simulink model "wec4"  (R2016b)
settings: Solver=ode4  StartTime=0  StopTime=1000  FixedStep=0.005  MaxStep=0.005  RelTol=1e-3  EnableMultiTasking=on
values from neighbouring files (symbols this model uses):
  arAdaptiveLawData = 1/2*zModelSimple.zModelPto.arFreq.*     zModelSimple.zModelPto.arMagnitude./     cos(zModelSimple.zModelPto.arPhase*pi/180+pi/2)    [IMPACT_Control.m]
  arAdaptiveLawDataX = 1/2*zModelSimpleX.zModelPto.arFreq.*         zModelSimpleX.zModelPto.arMagnitude./         cos(zModelSimpleX.zModelPto.arPhase*pi/180+pi/2)    [IMPACT_Control.m]
  arControllerRampGain = [0,0,1,1]    [IMPACT_Control.m]
  arControllerRampTime = [0 rStartRampTime rStartRampTime+rRampTimeLength 8000]    [IMPACT_Control.m]
  arEkfInitialisation = zeros(1,11)    [IMPACT_Control.m]
  arEkfInitialisationX = zeros(1,11)    [IMPACT_Control.m]
  arFrequency = zModelSimple.zModelPto.arFreq    [IMPACT_Control.m]
  arFrequencyRange = zModelSimple.zModelPto.arFreq    [IMPACT_Control.m]
  arFrequencyX = zModelSimpleX.zModelPto.arFreq    [IMPACT_Control.m]
  arImpedance = 1./zModelSimple.zModelPto.arMagnitude./zModelSimple.zModelPto.arFreq    [IMPACT_Control.m]
  arImpedanceX = 1./zModelSimpleX.zModelPto.arMagnitude./zModelSimpleX.zModelPto.arFreq    [IMPACT_Control.m]
  CentralPTOPreload = -1.6113e+07    (= -16113000)    [wecSimInputFile.m]
  F1 = [4.243 2.375 -12.243]    [wecSimInputFile.m]
  F2 = [4.243 -2.375 -12.243]    [wecSimInputFile.m]
  F3 = [-4.243 -2.375 -12.243]    [wecSimInputFile.m]
  F4 = [-4.243 2.375 -12.243]    [wecSimInputFile.m]
  FC = [0 0 -14]    [wecSimInputFile.m]
  iAdaptiveDamping = 0    [wec4IMPACT_Project.m]    (also in IMPACT_Control.m = handles.iAdaptiveDamping; wec1_IMPACT_Project.m; wec2_IMPACT_Project.m; wec3_IMPACT_Project.m)
  iControlType = 2    [wec4IMPACT_Project.m]    (also in IMPACT_Control.m = handles.iControlType; wec1_IMPACT_Project.m = 1; wec2_IMPACT_Project.m = 1; wec3_IMPACT_Project.m = 1)
  iPtoPositionConstraint = 1    [wec4IMPACT_Project.m]    (also in IMPACT_Control.m = handles.iPtoPositionConstraint; wec1_IMPACT_Project.m = 0; wec2_IMPACT_Project.m; wec3_IMPACT_Project.m)
  iSensorNoise = 0    [IMPACT_Control.m]
  m = m+1    (= 2)    [checkParamFile.m]
  PTOrotation = atan((T1(2)-F1(2))/(T1(1)-F1(1)))    [wecSimInputFile.m]
  rCogFloater = -8    [wec4_IMPACT_Model.m]    (also in paramInitial.m = get( handles.edit_rCogFloater, 'String' ); wec1_IMPACT_Model.m = -18; wec2_IMPACT_Model.m = -8.5; wec3_IMPACT_Model.m = -0.7)
  rCogSpar = -36.6    [wec4_IMPACT_Model.m]    (also in paramInitial.m = get( handles.edit_rCogSpar, 'String' ); wec3_IMPACT_Model.m = -21.3; wec3_IMPACT_Model2.m = -21.3)
  rDisplacementLimit = 10.000000    (= 10)    [wec4IMPACT_Project.m]    (also in IMPACT_Control.m = getValue(handles.edit_displacementLimit); wec1_IMPACT_Project.m; wec2_IMPACT_Project.m; wec3_IMPACT_Project.m = 3)
  rDisplacementLimitX = 10.000000    (= 10)    [wec4IMPACT_Project.m]    (also in IMPACT_Control.m = getValue(handles.edit_displacementLimitX); wec1_IMPACT_Project.m = 0; wec2_IMPACT_Project.m; wec3_IMPACT_Project.m = 0)
  rGainForAntiWIndUp = tfControllerDiscrete.rGain    [IMPACT_Control.m]
  rGainForAntiWIndUpX = tfControllerXDiscrete.rGain    [IMPACT_Control.m]
  rMaxForcePto = 300000000.000000    (= 300000000)    [wec4IMPACT_Project.m]    (also in IMPACT_Control.m = getValue(handles.edit_maxForcePto); wec1_IMPACT_Project.m = 1e+15; wec2_IMPACT_Project.m = 1e+15; wec3_IMPACT_Project.m = 1000000000)
  rMinForcePto = -300000000.000000    (= -300000000)    [wec4IMPACT_Project.m]    (also in IMPACT_Control.m = getValue(handles.edit_minForcePto); wec1_IMPACT_Project.m = -1e+15; wec2_IMPACT_Project.m = -1e+15; wec3_IMPACT_Project.m = -1000000000)
  rMooringX = 20000    [wec4_IMPACT_Model.m]    (also in paramInitial.m = get( handles.edit_rMooringX, 'String' ); wec3_IMPACT_Model.m = 10000; wec3_IMPACT_Model2.m = 10000)
  rMooringZ = 10000    [wec4_IMPACT_Model.m]    (also in paramInitial.m = get( handles.edit_rMooringZ, 'String' ); wec3_IMPACT_Model.m = 0; wec3_IMPACT_Model2.m = 0)
  rOutputSampleTime = 0.010000    (= 0.01)    [wec4IMPACT_Project.m]    (also in IMPACT_Control.m = getValue(handles.edit_outputSampleTime); wec1_IMPACT_Project.m; wec2_IMPACT_Project.m; wec3_IMPACT_Project.m)
  rPassiveDampingGain = -604830.000000    (= -604830)    [wec4IMPACT_Project.m]    (also in IMPACT_Control.m = getValue(handles.edit_gainPLD); wec1_IMPACT_Project.m = -214018.1537; wec2_IMPACT_Project.m = -1948070; wec3_IMPACT_Project.m = -519390)
  rPassiveDampingGainX = -278660.000000    (= -278660)    [wec4IMPACT_Project.m]    (also in IMPACT_Control.m = getValue(handles.edit_gainPLDX); wec1_IMPACT_Project.m = 0; wec2_IMPACT_Project.m = 0; wec3_IMPACT_Project.m = 0)
  rTetherPretension = 1.6113e+07    (= 16113000)    [wec4_IMPACT_Model.m]    (also in paramInitial.m = get( handles.edit_rTetherPretension, 'String' ); wec3_IMPACT_Model.m = 0; wec3_IMPACT_Model2.m = 0)
  rTetherSpring = 500000    [wec4_IMPACT_Model.m]    (also in paramInitial.m = get( handles.edit_rTetherSpring, 'String' ); wec3_IMPACT_Model.m = 0; wec3_IMPACT_Model2.m = 0)
  rUpperFrequencyLimit = EKFFloater.upperFreq    [IMPACT_Control.m]
  rXf = 4.243    [wec4AdditionalParams.m]
  rXs = 16.075    [wec4AdditionalParams.m]
  rYf = 2.375    [wec4AdditionalParams.m]
  rYs = 16.075    [wec4AdditionalParams.m]
  rZf = 4.243    [wec4AdditionalParams.m]
  rZs = 2.4350    (= 2.435)    [wec4AdditionalParams.m]
  rZTetherF = 6    [wec4AdditionalParams.m]
  rZTetherS = 2.4350    (= 2.435)    [wec4AdditionalParams.m]
  s = tf('s')    [wec4_IMPACT_Model.m]    (also in IMPACT_Control.m; wec1_IMPACT_Model.m; wec2_IMPACT_Model.m; wec3_IMPACT_Model.m)
  SidePTO1Preload = PreloadPTOCorner    (= 0)    [wecSimInputFile.m]
  SidePTO2Preload = PreloadPTOCorner    (= 0)    [wecSimInputFile.m]
  SidePTO3Preload = PreloadPTOCorner    (= 0)    [wecSimInputFile.m]
  SidePTO4Preload = PreloadPTOCorner    (= 0)    [wecSimInputFile.m]
  simu = simulationClass()    [wecSimInputFile.m]
  T1 = [16.075 16.075 -34.165]    [wecSimInputFile.m]
  T2 = [16.075 -16.075 -34.165]    [wecSimInputFile.m]
  T3 = [-16.075 -16.075 -34.165]    [wecSimInputFile.m]
  T4 = [-16.075 16.075 -34.165]    [wecSimInputFile.m]
  TC = [0 0 -34.165]    [wecSimInputFile.m]
  waves = waveClass('irregular')    [wecSimInputFile.m]
  Z = magPhaseToComplex(zModelTf)    [IMPACT_Control.m]
undefined symbols (not defined in the file or in its folder): arControllerDiscreteDen, arControllerDiscreteNum, arControllerDiscreteXDen, arControllerDiscreteXNum, arExcForceFloaterDen, arExcForceFloaterNum, arExcForceFloaterXDen, arExcForceFloaterXNum, arExcForceSparDen, arExcForceSparNum, arExcForceSparXDen, arExcForceSparXNum, arFexcFloaterDen, arFexcFloaterNum, arFexcFloaterXDen, arFexcFloaterXNum, arFexcSparDen, arFexcSparNum, arFexcSparXDen, arFexcSparXNum, Body, body, constraint, CTTime, deg, Elements, geometry, IRKB, kg, lenJ, mooring, N, pto, rAccelerationGainFloater, rAccelerationGainFloaterX, rAccelerationGainSpar, rAccelerationGainSparX, rad, rBuoyancyGainFloater, rBuoyancyGainFloaterX, rBuoyancyGainSpar, rBuoyancyGainSparX, rDampingGainFloater, rDampingGainFloaterX, rDampingGainSpar, rDampingGainSparX, Rigid, rMaxFocePto, wec4_float, wec4_reactor, WECSim_Lib, X, Y
libraries: nesl_utility x380, sm_lib x170, vrlib x91, simulink x12, WECSim_Lib x4
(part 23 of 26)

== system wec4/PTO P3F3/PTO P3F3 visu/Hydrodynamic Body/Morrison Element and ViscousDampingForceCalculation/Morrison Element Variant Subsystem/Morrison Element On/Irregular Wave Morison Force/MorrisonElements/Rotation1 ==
  rot1 : Inport
  rot2 : Inport  Port=2
  rot3 : Inport  Port=3
  2 : Product
  3 : Product  Inputs=3
  7 : Product
  8 : Product  Inputs=3
  Combine : Concatenate  NumInputs=3  Mode=Multidimensional array  ConcatenateDimension=2
  Trigonometric Function{,1..2,6,9,11} (6 alike) : Trigonometry  Operator=cos
  Trigonometric Function{3..5,7..8,10} (6 alike) : Trigonometry
  rot11 : Product
  rot12 : Sum
  rot13 : Sum  Inputs=+-
  rot[1,1-3] : Outport
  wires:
  rot13/1 -> Combine/3
  8/1 -> rot13/2
  7/1 -> rot13/1
  Trigonometric Function11/1 -> 8/3
  Trigonometric Function10/1 -> 8/2
  Trigonometric Function9/1 -> 8/1
  Trigonometric Function8/1 -> 7/2
  Trigonometric Function7/1 -> 7/1
  rot1/1 -> Trigonometric Function7/1, Trigonometric Function9/1, Trigonometric Function4/1, Trigonometric Function2/1
  rot3/1 -> Trigonometric Function8/1, Trigonometric Function11/1, Trigonometric Function6/1, Trigonometric Function3/1, Trigonometric Function1/1
  rot2/1 -> Trigonometric Function10/1, Trigonometric Function5/1, Trigonometric Function/1
  Combine/1 -> rot[1,1-3]/1
  rot12/1 -> Combine/2
  3/1 -> rot12/2
  2/1 -> rot12/1
  Trigonometric Function6/1 -> 3/3
  Trigonometric Function5/1 -> 3/2
  Trigonometric Function4/1 -> 3/1
  Trigonometric Function3/1 -> 2/2
  Trigonometric Function2/1 -> 2/1
  rot11/1 -> Combine/1
  Trigonometric Function1/1 -> rot11/2
  Trigonometric Function/1 -> rot11/1

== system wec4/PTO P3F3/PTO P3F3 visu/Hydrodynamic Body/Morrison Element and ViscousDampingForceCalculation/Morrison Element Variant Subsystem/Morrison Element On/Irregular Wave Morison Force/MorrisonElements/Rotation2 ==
  rot1 : Inport
  rot2 : Inport  Port=2
  rot3 : Inport  Port=3
  2 : Product
  3 : Product  Inputs=3
  7 : Product
  8 : Product  Inputs=3
  Combine : Concatenate  NumInputs=3  Mode=Multidimensional array  ConcatenateDimension=2
  Gain : Gain  Gain=-1
  Trigonometric Function{,2..3,8..9} (5 alike) : Trigonometry  Operator=cos
  Trigonometric Function{1,4..7,10..11} (7 alike) : Trigonometry
  rot11 : Product
  rot12 : Sum  Inputs=+-
  rot13 : Sum
  rot[2,1-3] : Outport
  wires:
  Gain/1 -> rot11/1
  rot13/1 -> Combine/3
  8/1 -> rot13/2
  7/1 -> rot13/1
  Trigonometric Function11/1 -> 8/3
  Trigonometric Function10/1 -> 8/2
  Trigonometric Function9/1 -> 8/1
  Trigonometric Function8/1 -> 7/2
  Trigonometric Function7/1 -> 7/1
  rot1/1 -> Trigonometric Function7/1, Trigonometric Function9/1, Trigonometric Function4/1, Trigonometric Function2/1
  rot3/1 -> Trigonometric Function8/1, Trigonometric Function11/1, Trigonometric Function6/1, Trigonometric Function3/1, Trigonometric Function1/1
  rot2/1 -> Trigonometric Function10/1, Trigonometric Function5/1, Trigonometric Function/1
  Combine/1 -> rot[2,1-3]/1
  rot12/1 -> Combine/2
  3/1 -> rot12/2
  2/1 -> rot12/1
  Trigonometric Function6/1 -> 3/3
  Trigonometric Function5/1 -> 3/2
  Trigonometric Function4/1 -> 3/1
  Trigonometric Function3/1 -> 2/2
  Trigonometric Function2/1 -> 2/1
  rot11/1 -> Combine/1
  Trigonometric Function1/1 -> rot11/2
  Trigonometric Function/1 -> Gain/1

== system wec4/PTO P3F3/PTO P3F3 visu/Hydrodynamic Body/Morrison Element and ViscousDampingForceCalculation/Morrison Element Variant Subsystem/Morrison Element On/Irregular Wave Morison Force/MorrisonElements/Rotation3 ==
  rot1 : Inport
  rot2 : Inport  Port=2
  2 : Product
  7 : Product
  Combine : Concatenate  NumInputs=3  Mode=Multidimensional array  ConcatenateDimension=2
  Gain1 : Gain  Gain=-1
  TrigFun1 : Trigonometry
  TrigFun2 : Trigonometry
  TrigFun3 : Trigonometry  Operator=cos
  TrigFun4 : Trigonometry  Operator=cos
  TrigFun5 : Trigonometry  Operator=cos
  rot[3,1-3] : Outport
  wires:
  Gain1/1 -> 2/1
  TrigFun2/1 -> Gain1/1
  7/1 -> Combine/3
  rot1/1 -> TrigFun4/1, TrigFun2/1
  TrigFun5/1 -> 7/2
  TrigFun4/1 -> 7/1
  rot2/1 -> TrigFun1/1, TrigFun3/1, TrigFun5/1
  Combine/1 -> rot[3,1-3]/1
  2/1 -> Combine/2
  TrigFun3/1 -> 2/2
  TrigFun1/1 -> Combine/1

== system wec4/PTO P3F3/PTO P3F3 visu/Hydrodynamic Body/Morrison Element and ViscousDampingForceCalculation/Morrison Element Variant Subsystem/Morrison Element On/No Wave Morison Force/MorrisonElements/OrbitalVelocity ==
  Disp : Inport
  Time : Inport  Port=2
  AmpMerge : Merge
  Applied Ramp Function : Subsystem  TreatAsAtomicUnit=on
  Disp-slx : Selector  InputPortWidth=3  IndexOptions=Index vector (dialog)  Indices=[1]  OutputSizes=1
  Disp-sly : Selector  InputPortWidth=3  IndexOptions=Index vector (dialog)  Indices=[2]  OutputSizes=1
  Disp-slz : Selector  InputPortWidth=3  IndexOptions=Index vector (dialog)  Indices=[3]  OutputSizes=1
  Gain : Gain  Gain=pi/180
  Gravity : Constant  Value=simu.g
  HorizHead : Trigonometry  Operator=cos
  Horizontal-x,y : Trigonometry  Operator=cos
  Horizontal-z : Trigonometry  Operator=cosh
  No Ramp Function : Subsystem  TreatAsAtomicUnit=on
  Ramp : If  NumInputs=2  IfExpression=u1 < u2
  Ramp Function Time : Constant  Value=simu.rampTime
  VertHead : Trigonometry
  Vertical-x,y : Trigonometry
  Vertical-z : Trigonometry  Operator=sinh
  WaterDepth : Constant  Value=waves.waterDepth
  WaveAmp : Constant  Value=waves.A(1,:)
  WaveFreq : Constant  Value=waves.w(1,:)
  WaveHeading : Constant  Value=waves.waveDir
  WaveNumber : Constant  Value=waves.k(1,:)
  X-A : Gain  Gain=-1
  Y-A : Gain  Gain=-1
  Y-V : Gain  Gain=-1
  Z-A : Gain  Gain=-1
  cosh : Trigonometry  Operator=cosh
  cosh*cos : Product  Inputs=**
  cosh*sin : Product  Inputs=**
  cosh/coshkh : Product  Inputs=*/
  k(xcos + ysin) : Sum
  k*h : Product
  k*x*cos(beta) : Product  Inputs=3
  k*y*sin(beta) : Product  Inputs=3
  k*z : Product
  sigma*t : Product
  sincos : Sum  Inputs=-+
  sinh*cos : Product  Inputs=**
  sinh*sin : Product  Inputs=**
  sinh/coshkh : Product  Inputs=*/
  sinhcosh : Sum
  u-Accel : Product  Inputs=*****
  u-Vel : Product  Inputs=****/*
  u-Vel1 : Product  Inputs=****/*
  v-Accel : Product  Inputs=*****
  w-Accel : Product  Inputs=****
  w-Vel : Product  Inputs=****/
  u-V : Outport
  w-V : Outport  Port=2
  u-A : Outport  Port=3
  w-A : Outport  Port=4
  v-V : Outport  Port=5
  v-A : Outport  Port=6
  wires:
  v-Accel/1 -> v-A/1
  Y-A/1 -> v-Accel/1
  u-Vel/1 -> u-V/1
  u-Vel1/1 -> v-V/1
  k(xcos + ysin)/1 -> sincos/1
  k*x*cos(beta)/1 -> k(xcos + ysin)/1
  k*y*sin(beta)/1 -> k(xcos + ysin)/2
  VertHead/1 -> v-Accel/5, u-Vel1/6, k*y*sin(beta)/1
  HorizHead/1 -> k*x*cos(beta)/1, u-Vel/6, u-Accel/5
  Disp-slx/1 -> k*x*cos(beta)/2
  Gain/1 -> VertHead/1, HorizHead/1
  WaveHeading/1 -> Gain/1
  WaveAmp/1 -> No Ramp Function/1(Ain), Applied Ramp Function/1(Ain)
  WaveFreq/1 -> sigma*t/1, u-Vel/5, u-Vel1/5, w-Vel/5
  Disp-slz/1 -> k*z/1
  Applied Ramp Function/1(Aout) -> AmpMerge/1
  No Ramp Function/1(Aout) -> AmpMerge/2
  Time/1 -> sigma*t/2, Ramp/1
  Ramp/1 -> Applied Ramp Function/Action
  Ramp/2 -> No Ramp Function/Action
  Ramp Function Time/1 -> Ramp/2
  sinh*cos/1 -> Z-A/1
  cosh*sin/1 -> X-A/1, Y-A/1
  w-Accel/1 -> w-A/1
  u-Accel/1 -> u-A/1
  w-Vel/1 -> w-V/1
  Z-A/1 -> w-Accel/1
  X-A/1 -> u-Accel/1
  Y-V/1 -> w-Vel/1
  sinh*sin/1 -> Y-V/1
  Gravity/1 -> u-Vel/3, u-Vel1/3, u-Accel/3, w-Accel/3, v-Accel/3, w-Vel/3
  AmpMerge/1 -> u-Vel/2, u-Vel1/2, u-Accel/2, v-Accel/2, w-Accel/2, w-Vel/2
  cosh*cos/1 -> u-Vel/1, u-Vel1/1
  Disp-sly/1 -> k*y*sin(beta)/2
  cosh/coshkh/1 -> cosh*sin/2, cosh*cos/2
  Horizontal-x,y/1 -> cosh*cos/1, sinh*cos/1
  sinh/coshkh/1 -> sinh*sin/2, sinh*cos/2
  Vertical-x,y/1 -> sinh*sin/1, cosh*sin/1
  Vertical-z/1 -> sinh/coshkh/1
  cosh/1 -> cosh/coshkh/2, sinh/coshkh/2
  Horizontal-z/1 -> cosh/coshkh/1
  sinhcosh/1 -> Horizontal-z/1, Vertical-z/1
  k*h/1 -> sinhcosh/2, cosh/1
  k*z/1 -> sinhcosh/1
  sincos/1 -> Horizontal-x,y/1, Vertical-x,y/1
  sigma*t/1 -> sincos/2
  WaterDepth/1 -> k*h/1
  WaveNumber/1 -> u-Vel/4, u-Vel1/4, u-Accel/4, w-Accel/4, v-Accel/4, w-Vel/4, k*x*cos(beta)/3, k*y*sin(beta)/3, k*z/2, k*h/2
  Disp/1 -> Disp-slx/1, Disp-sly/1, Disp-slz/1

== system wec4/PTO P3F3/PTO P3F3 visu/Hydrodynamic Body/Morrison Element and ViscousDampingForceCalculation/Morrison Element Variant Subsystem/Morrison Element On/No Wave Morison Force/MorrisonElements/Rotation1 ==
  rot1 : Inport
  rot2 : Inport  Port=2
  rot3 : Inport  Port=3
  2 : Product
  3 : Product  Inputs=3
  7 : Product
  8 : Product  Inputs=3
  Combine : Concatenate  NumInputs=3  Mode=Multidimensional array  ConcatenateDimension=2
  Trigonometric Function{,1..2,6,9,11} (6 alike) : Trigonometry  Operator=cos
  Trigonometric Function{3..5,7..8,10} (6 alike) : Trigonometry
  rot11 : Product
  rot12 : Sum
  rot13 : Sum  Inputs=+-
  rot[1,1-3] : Outport
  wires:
  rot13/1 -> Combine/3
  8/1 -> rot13/2
  7/1 -> rot13/1
  Trigonometric Function11/1 -> 8/3
  Trigonometric Function10/1 -> 8/2
  Trigonometric Function9/1 -> 8/1
  Trigonometric Function8/1 -> 7/2
  Trigonometric Function7/1 -> 7/1
  rot1/1 -> Trigonometric Function7/1, Trigonometric Function9/1, Trigonometric Function4/1, Trigonometric Function2/1
  rot3/1 -> Trigonometric Function8/1, Trigonometric Function11/1, Trigonometric Function6/1, Trigonometric Function3/1, Trigonometric Function1/1
  rot2/1 -> Trigonometric Function10/1, Trigonometric Function5/1, Trigonometric Function/1
  Combine/1 -> rot[1,1-3]/1
  rot12/1 -> Combine/2
  3/1 -> rot12/2
  2/1 -> rot12/1
  Trigonometric Function6/1 -> 3/3
  Trigonometric Function5/1 -> 3/2
  Trigonometric Function4/1 -> 3/1
  Trigonometric Function3/1 -> 2/2
  Trigonometric Function2/1 -> 2/1
  rot11/1 -> Combine/1
  Trigonometric Function1/1 -> rot11/2
  Trigonometric Function/1 -> rot11/1

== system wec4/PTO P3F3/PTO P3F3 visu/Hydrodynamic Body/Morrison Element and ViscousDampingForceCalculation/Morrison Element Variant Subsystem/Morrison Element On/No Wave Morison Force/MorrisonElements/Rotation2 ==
  rot1 : Inport
  rot2 : Inport  Port=2
  rot3 : Inport  Port=3
  2 : Product
  3 : Product  Inputs=3
  7 : Product
  8 : Product  Inputs=3
  Combine : Concatenate  NumInputs=3  Mode=Multidimensional array  ConcatenateDimension=2
  Gain : Gain  Gain=-1
  Trigonometric Function{,2..3,8..9} (5 alike) : Trigonometry  Operator=cos
  Trigonometric Function{1,4..7,10..11} (7 alike) : Trigonometry
  rot11 : Product
  rot12 : Sum  Inputs=+-
  rot13 : Sum
  rot[2,1-3] : Outport
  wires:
  Gain/1 -> rot11/1
  rot13/1 -> Combine/3
  8/1 -> rot13/2
  7/1 -> rot13/1
  Trigonometric Function11/1 -> 8/3
  Trigonometric Function10/1 -> 8/2
  Trigonometric Function9/1 -> 8/1
  Trigonometric Function8/1 -> 7/2
  Trigonometric Function7/1 -> 7/1
  rot1/1 -> Trigonometric Function7/1, Trigonometric Function9/1, Trigonometric Function4/1, Trigonometric Function2/1
  rot3/1 -> Trigonometric Function8/1, Trigonometric Function11/1, Trigonometric Function6/1, Trigonometric Function3/1, Trigonometric Function1/1
  rot2/1 -> Trigonometric Function10/1, Trigonometric Function5/1, Trigonometric Function/1
  Combine/1 -> rot[2,1-3]/1
  rot12/1 -> Combine/2
  3/1 -> rot12/2
  2/1 -> rot12/1
  Trigonometric Function6/1 -> 3/3
  Trigonometric Function5/1 -> 3/2
  Trigonometric Function4/1 -> 3/1
  Trigonometric Function3/1 -> 2/2
  Trigonometric Function2/1 -> 2/1
  rot11/1 -> Combine/1
  Trigonometric Function1/1 -> rot11/2
  Trigonometric Function/1 -> Gain/1

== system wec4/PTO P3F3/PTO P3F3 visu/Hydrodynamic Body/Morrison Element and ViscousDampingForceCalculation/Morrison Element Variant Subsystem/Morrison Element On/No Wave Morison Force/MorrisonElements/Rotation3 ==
  rot1 : Inport
  rot2 : Inport  Port=2
  2 : Product
  7 : Product
  Combine : Concatenate  NumInputs=3  Mode=Multidimensional array  ConcatenateDimension=2
  Gain1 : Gain  Gain=-1
  TrigFun1 : Trigonometry
  TrigFun2 : Trigonometry
  TrigFun3 : Trigonometry  Operator=cos
  TrigFun4 : Trigonometry  Operator=cos
  TrigFun5 : Trigonometry  Operator=cos
  rot[3,1-3] : Outport
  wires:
  Gain1/1 -> 2/1
  TrigFun2/1 -> Gain1/1
  7/1 -> Combine/3
  rot1/1 -> TrigFun4/1, TrigFun2/1
  TrigFun5/1 -> 7/2
  TrigFun4/1 -> 7/1
  rot2/1 -> TrigFun1/1, TrigFun3/1, TrigFun5/1
  Combine/1 -> rot[3,1-3]/1
  2/1 -> Combine/2
  TrigFun3/1 -> 2/2
  TrigFun1/1 -> Combine/1

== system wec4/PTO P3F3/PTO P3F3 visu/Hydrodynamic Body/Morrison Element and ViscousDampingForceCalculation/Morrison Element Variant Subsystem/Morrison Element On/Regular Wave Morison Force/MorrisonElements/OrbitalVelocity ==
  Disp : Inport
  Time : Inport  Port=2
  MATLAB Function : MATLAB Function  TreatAsAtomicUnit=on
  WaveAmp : Constant  Value=waves.A(1,:)
  WaveFreq : Constant  Value=waves.w(1,:)
  WaveNumber : Constant  Value=waves.k(1,:)
  gravity : Constant  Value=simu.g  VectorParams1D=off
  phase : Constant  Value=0
  rampTime : Constant  Value=simu.rampTime  VectorParams1D=off
  waterDepth : Constant  Value=waves.waterDepth  VectorParams1D=off
  waveDirection : Constant  Value=waves.waveDir  VectorParams1D=off
  u-V : Outport
  w-V : Outport  Port=2
  u-A : Outport  Port=3
  w-A : Outport  Port=4
  v-V : Outport  Port=5
  v-A : Outport  Port=6
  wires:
  MATLAB Function/5(ya) -> v-A/1
  MATLAB Function/1(u) -> u-V/1
  MATLAB Function/2(v) -> v-V/1
  MATLAB Function/6(za) -> w-A/1
  MATLAB Function/4(xa) -> u-A/1
  MATLAB Function/3(w) -> w-V/1
  rampTime/1 -> MATLAB Function/7(rampT)
  waveDirection/1 -> MATLAB Function/8(waveDir)
  waterDepth/1 -> MATLAB Function/9(waterDepth)
  gravity/1 -> MATLAB Function/10(g)
  Time/1 -> MATLAB Function/6(time)
  WaveAmp/1 -> MATLAB Function/4(waveAmp)
  WaveFreq/1 -> MATLAB Function/3(waveFreq)
  WaveNumber/1 -> MATLAB Function/2(waveNumber)
  phase/1 -> MATLAB Function/5(randPhase)
  Disp/1 -> MATLAB Function/1(disp)

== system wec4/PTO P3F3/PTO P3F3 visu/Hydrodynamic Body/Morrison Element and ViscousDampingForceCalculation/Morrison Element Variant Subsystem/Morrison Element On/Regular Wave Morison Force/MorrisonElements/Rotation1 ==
  rot1 : Inport
  rot2 : Inport  Port=2
  rot3 : Inport  Port=3
  2 : Product
  3 : Product  Inputs=3
  7 : Product
  8 : Product  Inputs=3
  Combine : Concatenate  NumInputs=3  Mode=Multidimensional array  ConcatenateDimension=2
  Trigonometric Function{,1..2,6,9,11} (6 alike) : Trigonometry  Operator=cos
  Trigonometric Function{3..5,7..8,10} (6 alike) : Trigonometry
  rot11 : Product
  rot12 : Sum
  rot13 : Sum  Inputs=+-
  rot[1,1-3] : Outport
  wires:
  rot13/1 -> Combine/3
  8/1 -> rot13/2
  7/1 -> rot13/1
  Trigonometric Function11/1 -> 8/3
  Trigonometric Function10/1 -> 8/2
  Trigonometric Function9/1 -> 8/1
  Trigonometric Function8/1 -> 7/2
  Trigonometric Function7/1 -> 7/1
  rot1/1 -> Trigonometric Function7/1, Trigonometric Function9/1, Trigonometric Function4/1, Trigonometric Function2/1
  rot3/1 -> Trigonometric Function8/1, Trigonometric Function11/1, Trigonometric Function6/1, Trigonometric Function3/1, Trigonometric Function1/1
  rot2/1 -> Trigonometric Function10/1, Trigonometric Function5/1, Trigonometric Function/1
  Combine/1 -> rot[1,1-3]/1
  rot12/1 -> Combine/2
  3/1 -> rot12/2
  2/1 -> rot12/1
  Trigonometric Function6/1 -> 3/3
  Trigonometric Function5/1 -> 3/2
  Trigonometric Function4/1 -> 3/1
  Trigonometric Function3/1 -> 2/2
  Trigonometric Function2/1 -> 2/1
  rot11/1 -> Combine/1
  Trigonometric Function1/1 -> rot11/2
  Trigonometric Function/1 -> rot11/1

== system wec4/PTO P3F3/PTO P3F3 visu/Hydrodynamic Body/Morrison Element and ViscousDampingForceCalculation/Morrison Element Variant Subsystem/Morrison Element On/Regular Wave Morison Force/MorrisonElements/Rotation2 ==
  rot1 : Inport
  rot2 : Inport  Port=2
  rot3 : Inport  Port=3
  2 : Product
  3 : Product  Inputs=3
  7 : Product
  8 : Product  Inputs=3
  Combine : Concatenate  NumInputs=3  Mode=Multidimensional array  ConcatenateDimension=2
  Gain : Gain  Gain=-1
  Trigonometric Function{,2..3,8..9} (5 alike) : Trigonometry  Operator=cos
  Trigonometric Function{1,4..7,10..11} (7 alike) : Trigonometry
  rot11 : Product
  rot12 : Sum  Inputs=+-
  rot13 : Sum
  rot[2,1-3] : Outport
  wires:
  Gain/1 -> rot11/1
  rot13/1 -> Combine/3
  8/1 -> rot13/2
  7/1 -> rot13/1
  Trigonometric Function11/1 -> 8/3
  Trigonometric Function10/1 -> 8/2
  Trigonometric Function9/1 -> 8/1
  Trigonometric Function8/1 -> 7/2
  Trigonometric Function7/1 -> 7/1
  rot1/1 -> Trigonometric Function7/1, Trigonometric Function9/1, Trigonometric Function4/1, Trigonometric Function2/1
  rot3/1 -> Trigonometric Function8/1, Trigonometric Function11/1, Trigonometric Function6/1, Trigonometric Function3/1, Trigonometric Function1/1
  rot2/1 -> Trigonometric Function10/1, Trigonometric Function5/1, Trigonometric Function/1
  Combine/1 -> rot[2,1-3]/1
  rot12/1 -> Combine/2
  3/1 -> rot12/2
  2/1 -> rot12/1
  Trigonometric Function6/1 -> 3/3
  Trigonometric Function5/1 -> 3/2
  Trigonometric Function4/1 -> 3/1
  Trigonometric Function3/1 -> 2/2
  Trigonometric Function2/1 -> 2/1
  rot11/1 -> Combine/1
  Trigonometric Function1/1 -> rot11/2
  Trigonometric Function/1 -> Gain/1

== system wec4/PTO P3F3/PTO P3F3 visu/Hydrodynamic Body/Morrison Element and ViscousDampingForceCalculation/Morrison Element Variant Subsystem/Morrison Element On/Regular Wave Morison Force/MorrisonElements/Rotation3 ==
  rot1 : Inport
  rot2 : Inport  Port=2
  2 : Product
  7 : Product
  Combine : Concatenate  NumInputs=3  Mode=Multidimensional array  ConcatenateDimension=2
  Gain1 : Gain  Gain=-1
  TrigFun1 : Trigonometry
  TrigFun2 : Trigonometry
  TrigFun3 : Trigonometry  Operator=cos
  TrigFun4 : Trigonometry  Operator=cos
  TrigFun5 : Trigonometry  Operator=cos
  rot[3,1-3] : Outport
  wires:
  Gain1/1 -> 2/1
  TrigFun2/1 -> Gain1/1
  7/1 -> Combine/3
  rot1/1 -> TrigFun4/1, TrigFun2/1
  TrigFun5/1 -> 7/2
  TrigFun4/1 -> 7/1
  rot2/1 -> TrigFun1/1, TrigFun3/1, TrigFun5/1
  Combine/1 -> rot[3,1-3]/1
  2/1 -> Combine/2
  TrigFun3/1 -> 2/2
  TrigFun1/1 -> Combine/1

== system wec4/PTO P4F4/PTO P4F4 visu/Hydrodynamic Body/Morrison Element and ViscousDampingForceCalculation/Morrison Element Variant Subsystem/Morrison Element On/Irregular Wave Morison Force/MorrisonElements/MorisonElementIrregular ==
  Disp : Inport
  waves.kirr : Inport  Port=2  Partition=on  PartitionDimension=1  PartitionWidth=1
  waves.w : Inport  Port=3  Partition=on  PartitionDimension=1  PartitionWidth=1
  waves.A : Inport  Port=4  Partition=on  PartitionDimension=1  PartitionWidth=1
  waves.Phase : Inport  Port=5  Partition=on  PartitionDimension=1  PartitionWidth=1
  Time : Inport  Port=6
  For Each : ForEach  DisableCoverage=on  IndexMode=One-based
  MATLAB Function : MATLAB Function  TreatAsAtomicUnit=on
  gravity : Constant  Value=simu.g  VectorParams1D=off
  rampTime : Constant  Value=simu.rampTime  VectorParams1D=off
  waterDepth : Constant  Value=waves.waterDepth  VectorParams1D=off
  waveDirection : Constant  Value=waves.waveDir  VectorParams1D=off
  u-V : Outport  ConcatenationDimension=1
  w-V : Outport  Port=2  ConcatenationDimension=1
  x-A : Outport  Port=3  ConcatenationDimension=1
  w-A : Outport  Port=4  ConcatenationDimension=1
  v-V : Outport  Port=5  ConcatenationDimension=1
  y-A : Outport  Port=6  ConcatenationDimension=1
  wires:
  MATLAB Function/3(w) -> w-V/1
  MATLAB Function/4(xa) -> x-A/1
  MATLAB Function/6(za) -> w-A/1
  MATLAB Function/5(ya) -> y-A/1
  MATLAB Function/2(v) -> v-V/1
  Time/1 -> MATLAB Function/6(time)
  waves.kirr/1 -> MATLAB Function/2(waveNumber)
  MATLAB Function/1(u) -> u-V/1
  waves.Phase/1 -> MATLAB Function/5(phase)
  waves.A/1 -> MATLAB Function/4(waveAmp)
  waves.w/1 -> MATLAB Function/3(waveFreq)
  Disp/1 -> MATLAB Function/1(disp)
  rampTime/1 -> MATLAB Function/7(rampT)
  waveDirection/1 -> MATLAB Function/8(waveDir)
  waterDepth/1 -> MATLAB Function/9(waterDepth)
  gravity/1 -> MATLAB Function/10(g)

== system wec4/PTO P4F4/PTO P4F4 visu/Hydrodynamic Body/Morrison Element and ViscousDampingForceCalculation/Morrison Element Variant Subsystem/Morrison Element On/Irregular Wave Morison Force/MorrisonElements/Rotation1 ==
  rot1 : Inport
  rot2 : Inport  Port=2
  rot3 : Inport  Port=3
  2 : Product
  3 : Product  Inputs=3
  7 : Product
  8 : Product  Inputs=3
  Combine : Concatenate  NumInputs=3  Mode=Multidimensional array  ConcatenateDimension=2
  Trigonometric Function{,1..2,6,9,11} (6 alike) : Trigonometry  Operator=cos
  Trigonometric Function{3..5,7..8,10} (6 alike) : Trigonometry
  rot11 : Product
  rot12 : Sum
  rot13 : Sum  Inputs=+-
  rot[1,1-3] : Outport
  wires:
  rot13/1 -> Combine/3
  8/1 -> rot13/2
  7/1 -> rot13/1
  Trigonometric Function11/1 -> 8/3
  Trigonometric Function10/1 -> 8/2
  Trigonometric Function9/1 -> 8/1
  Trigonometric Function8/1 -> 7/2
  Trigonometric Function7/1 -> 7/1
  rot1/1 -> Trigonometric Function7/1, Trigonometric Function9/1, Trigonometric Function4/1, Trigonometric Function2/1
  rot3/1 -> Trigonometric Function8/1, Trigonometric Function11/1, Trigonometric Function6/1, Trigonometric Function3/1, Trigonometric Function1/1
  rot2/1 -> Trigonometric Function10/1, Trigonometric Function5/1, Trigonometric Function/1
  Combine/1 -> rot[1,1-3]/1
  rot12/1 -> Combine/2
  3/1 -> rot12/2
  2/1 -> rot12/1
  Trigonometric Function6/1 -> 3/3
  Trigonometric Function5/1 -> 3/2
  Trigonometric Function4/1 -> 3/1
  Trigonometric Function3/1 -> 2/2
  Trigonometric Function2/1 -> 2/1
  rot11/1 -> Combine/1
  Trigonometric Function1/1 -> rot11/2
  Trigonometric Function/1 -> rot11/1

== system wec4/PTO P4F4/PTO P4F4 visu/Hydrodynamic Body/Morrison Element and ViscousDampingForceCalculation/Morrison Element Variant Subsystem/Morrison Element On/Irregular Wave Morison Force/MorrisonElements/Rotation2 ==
  rot1 : Inport
  rot2 : Inport  Port=2
  rot3 : Inport  Port=3
  2 : Product
  3 : Product  Inputs=3
  7 : Product
  8 : Product  Inputs=3
  Combine : Concatenate  NumInputs=3  Mode=Multidimensional array  ConcatenateDimension=2
  Gain : Gain  Gain=-1
  Trigonometric Function{,2..3,8..9} (5 alike) : Trigonometry  Operator=cos
  Trigonometric Function{1,4..7,10..11} (7 alike) : Trigonometry
  rot11 : Product
  rot12 : Sum  Inputs=+-
  rot13 : Sum
  rot[2,1-3] : Outport
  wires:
  Gain/1 -> rot11/1
  rot13/1 -> Combine/3
  8/1 -> rot13/2
  7/1 -> rot13/1
  Trigonometric Function11/1 -> 8/3
  Trigonometric Function10/1 -> 8/2
  Trigonometric Function9/1 -> 8/1
  Trigonometric Function8/1 -> 7/2
  Trigonometric Function7/1 -> 7/1
  rot1/1 -> Trigonometric Function7/1, Trigonometric Function9/1, Trigonometric Function4/1, Trigonometric Function2/1
  rot3/1 -> Trigonometric Function8/1, Trigonometric Function11/1, Trigonometric Function6/1, Trigonometric Function3/1, Trigonometric Function1/1
  rot2/1 -> Trigonometric Function10/1, Trigonometric Function5/1, Trigonometric Function/1
  Combine/1 -> rot[2,1-3]/1
  rot12/1 -> Combine/2
  3/1 -> rot12/2
  2/1 -> rot12/1
  Trigonometric Function6/1 -> 3/3
  Trigonometric Function5/1 -> 3/2
  Trigonometric Function4/1 -> 3/1
  Trigonometric Function3/1 -> 2/2
  Trigonometric Function2/1 -> 2/1
  rot11/1 -> Combine/1
  Trigonometric Function1/1 -> rot11/2
  Trigonometric Function/1 -> Gain/1

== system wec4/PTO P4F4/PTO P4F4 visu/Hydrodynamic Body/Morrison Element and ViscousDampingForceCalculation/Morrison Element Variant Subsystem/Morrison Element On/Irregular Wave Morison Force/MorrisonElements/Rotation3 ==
  rot1 : Inport
  rot2 : Inport  Port=2
  2 : Product
  7 : Product
  Combine : Concatenate  NumInputs=3  Mode=Multidimensional array  ConcatenateDimension=2
  Gain1 : Gain  Gain=-1
  TrigFun1 : Trigonometry
  TrigFun2 : Trigonometry
  TrigFun3 : Trigonometry  Operator=cos
  TrigFun4 : Trigonometry  Operator=cos
  TrigFun5 : Trigonometry  Operator=cos
  rot[3,1-3] : Outport
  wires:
  Gain1/1 -> 2/1
  TrigFun2/1 -> Gain1/1
  7/1 -> Combine/3
  rot1/1 -> TrigFun4/1, TrigFun2/1
  TrigFun5/1 -> 7/2
  TrigFun4/1 -> 7/1
  rot2/1 -> TrigFun1/1, TrigFun3/1, TrigFun5/1
  Combine/1 -> rot[3,1-3]/1
  2/1 -> Combine/2
  TrigFun3/1 -> 2/2
  TrigFun1/1 -> Combine/1

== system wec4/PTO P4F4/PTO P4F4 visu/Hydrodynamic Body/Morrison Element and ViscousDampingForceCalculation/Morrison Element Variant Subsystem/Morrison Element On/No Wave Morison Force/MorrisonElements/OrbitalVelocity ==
  Disp : Inport
  Time : Inport  Port=2
  AmpMerge : Merge
  Applied Ramp Function : Subsystem  TreatAsAtomicUnit=on
  Disp-slx : Selector  InputPortWidth=3  IndexOptions=Index vector (dialog)  Indices=[1]  OutputSizes=1
  Disp-sly : Selector  InputPortWidth=3  IndexOptions=Index vector (dialog)  Indices=[2]  OutputSizes=1
  Disp-slz : Selector  InputPortWidth=3  IndexOptions=Index vector (dialog)  Indices=[3]  OutputSizes=1
  Gain : Gain  Gain=pi/180
  Gravity : Constant  Value=simu.g
  HorizHead : Trigonometry  Operator=cos
  Horizontal-x,y : Trigonometry  Operator=cos
  Horizontal-z : Trigonometry  Operator=cosh
  No Ramp Function : Subsystem  TreatAsAtomicUnit=on
  Ramp : If  NumInputs=2  IfExpression=u1 < u2
  Ramp Function Time : Constant  Value=simu.rampTime
  VertHead : Trigonometry
  Vertical-x,y : Trigonometry
  Vertical-z : Trigonometry  Operator=sinh
  WaterDepth : Constant  Value=waves.waterDepth
  WaveAmp : Constant  Value=waves.A(1,:)
  WaveFreq : Constant  Value=waves.w(1,:)
  WaveHeading : Constant  Value=waves.waveDir
  WaveNumber : Constant  Value=waves.k(1,:)
  X-A : Gain  Gain=-1
  Y-A : Gain  Gain=-1
  Y-V : Gain  Gain=-1
  Z-A : Gain  Gain=-1
  cosh : Trigonometry  Operator=cosh
  cosh*cos : Product  Inputs=**
  cosh*sin : Product  Inputs=**
  cosh/coshkh : Product  Inputs=*/
  k(xcos + ysin) : Sum
  k*h : Product
  k*x*cos(beta) : Product  Inputs=3
  k*y*sin(beta) : Product  Inputs=3
  k*z : Product
  sigma*t : Product
  sincos : Sum  Inputs=-+
  sinh*cos : Product  Inputs=**
  sinh*sin : Product  Inputs=**
  sinh/coshkh : Product  Inputs=*/
  sinhcosh : Sum
  u-Accel : Product  Inputs=*****
  u-Vel : Product  Inputs=****/*
  u-Vel1 : Product  Inputs=****/*
  v-Accel : Product  Inputs=*****
  w-Accel : Product  Inputs=****
  w-Vel : Product  Inputs=****/
  u-V : Outport
  w-V : Outport  Port=2
  u-A : Outport  Port=3
  w-A : Outport  Port=4
  v-V : Outport  Port=5
  v-A : Outport  Port=6
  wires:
  v-Accel/1 -> v-A/1
  Y-A/1 -> v-Accel/1
  u-Vel/1 -> u-V/1
  u-Vel1/1 -> v-V/1
  k(xcos + ysin)/1 -> sincos/1
  k*x*cos(beta)/1 -> k(xcos + ysin)/1
  k*y*sin(beta)/1 -> k(xcos + ysin)/2
  VertHead/1 -> v-Accel/5, u-Vel1/6, k*y*sin(beta)/1
  HorizHead/1 -> k*x*cos(beta)/1, u-Vel/6, u-Accel/5
  Disp-slx/1 -> k*x*cos(beta)/2
  Gain/1 -> VertHead/1, HorizHead/1
  WaveHeading/1 -> Gain/1
  WaveAmp/1 -> No Ramp Function/1(Ain), Applied Ramp Function/1(Ain)
  WaveFreq/1 -> sigma*t/1, u-Vel/5, u-Vel1/5, w-Vel/5
  Disp-slz/1 -> k*z/1
  Applied Ramp Function/1(Aout) -> AmpMerge/1
  No Ramp Function/1(Aout) -> AmpMerge/2
  Time/1 -> sigma*t/2, Ramp/1
  Ramp/1 -> Applied Ramp Function/Action
  Ramp/2 -> No Ramp Function/Action
  Ramp Function Time/1 -> Ramp/2
  sinh*cos/1 -> Z-A/1
  cosh*sin/1 -> X-A/1, Y-A/1
  w-Accel/1 -> w-A/1
  u-Accel/1 -> u-A/1
  w-Vel/1 -> w-V/1
  Z-A/1 -> w-Accel/1
  X-A/1 -> u-Accel/1
  Y-V/1 -> w-Vel/1
  sinh*sin/1 -> Y-V/1
  Gravity/1 -> u-Vel/3, u-Vel1/3, u-Accel/3, w-Accel/3, v-Accel/3, w-Vel/3
  AmpMerge/1 -> u-Vel/2, u-Vel1/2, u-Accel/2, v-Accel/2, w-Accel/2, w-Vel/2
  cosh*cos/1 -> u-Vel/1, u-Vel1/1
  Disp-sly/1 -> k*y*sin(beta)/2
  cosh/coshkh/1 -> cosh*sin/2, cosh*cos/2
  Horizontal-x,y/1 -> cosh*cos/1, sinh*cos/1
  sinh/coshkh/1 -> sinh*sin/2, sinh*cos/2
  Vertical-x,y/1 -> sinh*sin/1, cosh*sin/1
  Vertical-z/1 -> sinh/coshkh/1
  cosh/1 -> cosh/coshkh/2, sinh/coshkh/2
  Horizontal-z/1 -> cosh/coshkh/1
  sinhcosh/1 -> Horizontal-z/1, Vertical-z/1
  k*h/1 -> sinhcosh/2, cosh/1
  k*z/1 -> sinhcosh/1
  sincos/1 -> Horizontal-x,y/1, Vertical-x,y/1
  sigma*t/1 -> sincos/2
  WaterDepth/1 -> k*h/1
  WaveNumber/1 -> u-Vel/4, u-Vel1/4, u-Accel/4, w-Accel/4, v-Accel/4, w-Vel/4, k*x*cos(beta)/3, k*y*sin(beta)/3, k*z/2, k*h/2
  Disp/1 -> Disp-slx/1, Disp-sly/1, Disp-slz/1

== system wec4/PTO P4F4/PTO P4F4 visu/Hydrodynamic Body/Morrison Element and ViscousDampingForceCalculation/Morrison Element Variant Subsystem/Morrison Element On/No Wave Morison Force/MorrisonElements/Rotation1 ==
  rot1 : Inport
  rot2 : Inport  Port=2
  rot3 : Inport  Port=3
  2 : Product
  3 : Product  Inputs=3
  7 : Product
  8 : Product  Inputs=3
  Combine : Concatenate  NumInputs=3  Mode=Multidimensional array  ConcatenateDimension=2
  Trigonometric Function{,1..2,6,9,11} (6 alike) : Trigonometry  Operator=cos
  Trigonometric Function{3..5,7..8,10} (6 alike) : Trigonometry
  rot11 : Product
  rot12 : Sum
  rot13 : Sum  Inputs=+-
  rot[1,1-3] : Outport
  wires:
  rot13/1 -> Combine/3
  8/1 -> rot13/2
  7/1 -> rot13/1
  Trigonometric Function11/1 -> 8/3
  Trigonometric Function10/1 -> 8/2
  Trigonometric Function9/1 -> 8/1
  Trigonometric Function8/1 -> 7/2
  Trigonometric Function7/1 -> 7/1
  rot1/1 -> Trigonometric Function7/1, Trigonometric Function9/1, Trigonometric Function4/1, Trigonometric Function2/1
  rot3/1 -> Trigonometric Function8/1, Trigonometric Function11/1, Trigonometric Function6/1, Trigonometric Function3/1, Trigonometric Function1/1
  rot2/1 -> Trigonometric Function10/1, Trigonometric Function5/1, Trigonometric Function/1
  Combine/1 -> rot[1,1-3]/1
  rot12/1 -> Combine/2
  3/1 -> rot12/2
  2/1 -> rot12/1
  Trigonometric Function6/1 -> 3/3
  Trigonometric Function5/1 -> 3/2
  Trigonometric Function4/1 -> 3/1
  Trigonometric Function3/1 -> 2/2
  Trigonometric Function2/1 -> 2/1
  rot11/1 -> Combine/1
  Trigonometric Function1/1 -> rot11/2
  Trigonometric Function/1 -> rot11/1

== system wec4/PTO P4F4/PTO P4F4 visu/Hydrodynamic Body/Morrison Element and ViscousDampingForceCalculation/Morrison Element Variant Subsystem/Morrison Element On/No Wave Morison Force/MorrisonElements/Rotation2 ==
  rot1 : Inport
  rot2 : Inport  Port=2
  rot3 : Inport  Port=3
  2 : Product
  3 : Product  Inputs=3
  7 : Product
  8 : Product  Inputs=3
  Combine : Concatenate  NumInputs=3  Mode=Multidimensional array  ConcatenateDimension=2
  Gain : Gain  Gain=-1
  Trigonometric Function{,2..3,8..9} (5 alike) : Trigonometry  Operator=cos
  Trigonometric Function{1,4..7,10..11} (7 alike) : Trigonometry
  rot11 : Product
  rot12 : Sum  Inputs=+-
  rot13 : Sum
  rot[2,1-3] : Outport
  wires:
  Gain/1 -> rot11/1
  rot13/1 -> Combine/3
  8/1 -> rot13/2
  7/1 -> rot13/1
  Trigonometric Function11/1 -> 8/3
  Trigonometric Function10/1 -> 8/2
  Trigonometric Function9/1 -> 8/1
  Trigonometric Function8/1 -> 7/2
  Trigonometric Function7/1 -> 7/1
  rot1/1 -> Trigonometric Function7/1, Trigonometric Function9/1, Trigonometric Function4/1, Trigonometric Function2/1
  rot3/1 -> Trigonometric Function8/1, Trigonometric Function11/1, Trigonometric Function6/1, Trigonometric Function3/1, Trigonometric Function1/1
  rot2/1 -> Trigonometric Function10/1, Trigonometric Function5/1, Trigonometric Function/1
  Combine/1 -> rot[2,1-3]/1
  rot12/1 -> Combine/2
  3/1 -> rot12/2
  2/1 -> rot12/1
  Trigonometric Function6/1 -> 3/3
  Trigonometric Function5/1 -> 3/2
  Trigonometric Function4/1 -> 3/1
  Trigonometric Function3/1 -> 2/2
  Trigonometric Function2/1 -> 2/1
  rot11/1 -> Combine/1
  Trigonometric Function1/1 -> rot11/2
  Trigonometric Function/1 -> Gain/1

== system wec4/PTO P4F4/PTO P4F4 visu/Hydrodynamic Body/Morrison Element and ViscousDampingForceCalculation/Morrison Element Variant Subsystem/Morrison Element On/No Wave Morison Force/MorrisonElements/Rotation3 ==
  rot1 : Inport
  rot2 : Inport  Port=2
  2 : Product
  7 : Product
  Combine : Concatenate  NumInputs=3  Mode=Multidimensional array  ConcatenateDimension=2
  Gain1 : Gain  Gain=-1
  TrigFun1 : Trigonometry
  TrigFun2 : Trigonometry
  TrigFun3 : Trigonometry  Operator=cos
  TrigFun4 : Trigonometry  Operator=cos
  TrigFun5 : Trigonometry  Operator=cos
  rot[3,1-3] : Outport
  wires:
  Gain1/1 -> 2/1
  TrigFun2/1 -> Gain1/1
  7/1 -> Combine/3
  rot1/1 -> TrigFun4/1, TrigFun2/1
  TrigFun5/1 -> 7/2
  TrigFun4/1 -> 7/1
  rot2/1 -> TrigFun1/1, TrigFun3/1, TrigFun5/1
  Combine/1 -> rot[3,1-3]/1
  2/1 -> Combine/2
  TrigFun3/1 -> 2/2
  TrigFun1/1 -> Combine/1

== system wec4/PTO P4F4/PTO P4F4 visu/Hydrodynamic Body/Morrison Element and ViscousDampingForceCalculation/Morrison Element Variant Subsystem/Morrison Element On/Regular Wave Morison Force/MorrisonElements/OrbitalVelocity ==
  Disp : Inport
  Time : Inport  Port=2
  MATLAB Function : MATLAB Function  TreatAsAtomicUnit=on
  WaveAmp : Constant  Value=waves.A(1,:)
  WaveFreq : Constant  Value=waves.w(1,:)
  WaveNumber : Constant  Value=waves.k(1,:)
  gravity : Constant  Value=simu.g  VectorParams1D=off
  phase : Constant  Value=0
  rampTime : Constant  Value=simu.rampTime  VectorParams1D=off
  waterDepth : Constant  Value=waves.waterDepth  VectorParams1D=off
  waveDirection : Constant  Value=waves.waveDir  VectorParams1D=off
  u-V : Outport
  w-V : Outport  Port=2
  u-A : Outport  Port=3
  w-A : Outport  Port=4
  v-V : Outport  Port=5
  v-A : Outport  Port=6
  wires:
  MATLAB Function/5(ya) -> v-A/1
  MATLAB Function/1(u) -> u-V/1
  MATLAB Function/2(v) -> v-V/1
  MATLAB Function/6(za) -> w-A/1
  MATLAB Function/4(xa) -> u-A/1
  MATLAB Function/3(w) -> w-V/1
  rampTime/1 -> MATLAB Function/7(rampT)
  waveDirection/1 -> MATLAB Function/8(waveDir)
  waterDepth/1 -> MATLAB Function/9(waterDepth)
  gravity/1 -> MATLAB Function/10(g)
  Time/1 -> MATLAB Function/6(time)
  WaveAmp/1 -> MATLAB Function/4(waveAmp)
  WaveFreq/1 -> MATLAB Function/3(waveFreq)
  WaveNumber/1 -> MATLAB Function/2(waveNumber)
  phase/1 -> MATLAB Function/5(randPhase)
  Disp/1 -> MATLAB Function/1(disp)

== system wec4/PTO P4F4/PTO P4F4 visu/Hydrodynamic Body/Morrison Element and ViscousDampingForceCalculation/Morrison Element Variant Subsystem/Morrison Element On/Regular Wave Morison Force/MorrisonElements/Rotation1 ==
  rot1 : Inport
  rot2 : Inport  Port=2
  rot3 : Inport  Port=3
  2 : Product
  3 : Product  Inputs=3
  7 : Product
  8 : Product  Inputs=3
  Combine : Concatenate  NumInputs=3  Mode=Multidimensional array  ConcatenateDimension=2
  Trigonometric Function{,1..2,6,9,11} (6 alike) : Trigonometry  Operator=cos
  Trigonometric Function{3..5,7..8,10} (6 alike) : Trigonometry
  rot11 : Product
  rot12 : Sum
  rot13 : Sum  Inputs=+-
  rot[1,1-3] : Outport
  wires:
  rot13/1 -> Combine/3
  8/1 -> rot13/2
  7/1 -> rot13/1
  Trigonometric Function11/1 -> 8/3
  Trigonometric Function10/1 -> 8/2
  Trigonometric Function9/1 -> 8/1
  Trigonometric Function8/1 -> 7/2
  Trigonometric Function7/1 -> 7/1
  rot1/1 -> Trigonometric Function7/1, Trigonometric Function9/1, Trigonometric Function4/1, Trigonometric Function2/1
  rot3/1 -> Trigonometric Function8/1, Trigonometric Function11/1, Trigonometric Function6/1, Trigonometric Function3/1, Trigonometric Function1/1
  rot2/1 -> Trigonometric Function10/1, Trigonometric Function5/1, Trigonometric Function/1
  Combine/1 -> rot[1,1-3]/1
  rot12/1 -> Combine/2
  3/1 -> rot12/2
  2/1 -> rot12/1
  Trigonometric Function6/1 -> 3/3
  Trigonometric Function5/1 -> 3/2
  Trigonometric Function4/1 -> 3/1
  Trigonometric Function3/1 -> 2/2
  Trigonometric Function2/1 -> 2/1
  rot11/1 -> Combine/1
  Trigonometric Function1/1 -> rot11/2
  Trigonometric Function/1 -> rot11/1

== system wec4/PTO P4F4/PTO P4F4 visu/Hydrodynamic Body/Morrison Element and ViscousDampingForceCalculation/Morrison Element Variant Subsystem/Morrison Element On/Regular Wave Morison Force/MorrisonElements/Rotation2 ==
  rot1 : Inport
  rot2 : Inport  Port=2
  rot3 : Inport  Port=3
  2 : Product
  3 : Product  Inputs=3
  7 : Product
  8 : Product  Inputs=3
  Combine : Concatenate  NumInputs=3  Mode=Multidimensional array  ConcatenateDimension=2
  Gain : Gain  Gain=-1
  Trigonometric Function{,2..3,8..9} (5 alike) : Trigonometry  Operator=cos
  Trigonometric Function{1,4..7,10..11} (7 alike) : Trigonometry
  rot11 : Product
  rot12 : Sum  Inputs=+-
  rot13 : Sum
  rot[2,1-3] : Outport
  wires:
  Gain/1 -> rot11/1
  rot13/1 -> Combine/3
  8/1 -> rot13/2
  7/1 -> rot13/1
  Trigonometric Function11/1 -> 8/3
  Trigonometric Function10/1 -> 8/2
  Trigonometric Function9/1 -> 8/1
  Trigonometric Function8/1 -> 7/2
  Trigonometric Function7/1 -> 7/1
  rot1/1 -> Trigonometric Function7/1, Trigonometric Function9/1, Trigonometric Function4/1, Trigonometric Function2/1
  rot3/1 -> Trigonometric Function8/1, Trigonometric Function11/1, Trigonometric Function6/1, Trigonometric Function3/1, Trigonometric Function1/1
  rot2/1 -> Trigonometric Function10/1, Trigonometric Function5/1, Trigonometric Function/1
  Combine/1 -> rot[2,1-3]/1
  rot12/1 -> Combine/2
  3/1 -> rot12/2
  2/1 -> rot12/1
  Trigonometric Function6/1 -> 3/3
  Trigonometric Function5/1 -> 3/2
  Trigonometric Function4/1 -> 3/1
  Trigonometric Function3/1 -> 2/2
  Trigonometric Function2/1 -> 2/1
  rot11/1 -> Combine/1
  Trigonometric Function1/1 -> rot11/2
  Trigonometric Function/1 -> Gain/1

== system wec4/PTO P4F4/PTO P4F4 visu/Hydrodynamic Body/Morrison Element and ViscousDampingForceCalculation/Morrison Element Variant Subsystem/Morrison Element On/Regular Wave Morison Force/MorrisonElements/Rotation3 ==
  rot1 : Inport
  rot2 : Inport  Port=2
  2 : Product
  7 : Product
  Combine : Concatenate  NumInputs=3  Mode=Multidimensional array  ConcatenateDimension=2
  Gain1 : Gain  Gain=-1
  TrigFun1 : Trigonometry
  TrigFun2 : Trigonometry
  TrigFun3 : Trigonometry  Operator=cos
  TrigFun4 : Trigonometry  Operator=cos
  TrigFun5 : Trigonometry  Operator=cos
  rot[3,1-3] : Outport
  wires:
  Gain1/1 -> 2/1
  TrigFun2/1 -> Gain1/1
  7/1 -> Combine/3
  rot1/1 -> TrigFun4/1, TrigFun2/1
  TrigFun5/1 -> 7/2
  TrigFun4/1 -> 7/1
  rot2/1 -> TrigFun1/1, TrigFun3/1, TrigFun5/1
  Combine/1 -> rot[3,1-3]/1
  2/1 -> Combine/2
  TrigFun3/1 -> 2/2
  TrigFun1/1 -> Combine/1

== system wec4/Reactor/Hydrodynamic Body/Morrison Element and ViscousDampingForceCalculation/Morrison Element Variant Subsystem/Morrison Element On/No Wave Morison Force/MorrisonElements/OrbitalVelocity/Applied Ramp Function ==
  Ain : Inport
  Action Port : ActionPort
  Add : Sum
  Constant : Constant  Value=2
  Constant1 : Constant
  Divide : Product  Inputs=**/
  Sine Wave : Sin  Frequency=pi/simu.rampTime  Phase=pi+pi/2  SampleTime=0
  Aout : Outport
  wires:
  Add/1 -> Divide/2
  Sine Wave/1 -> Add/2
  Constant1/1 -> Add/1
  Constant/1 -> Divide/3
  Divide/1 -> Aout/1
  Ain/1 -> Divide/1

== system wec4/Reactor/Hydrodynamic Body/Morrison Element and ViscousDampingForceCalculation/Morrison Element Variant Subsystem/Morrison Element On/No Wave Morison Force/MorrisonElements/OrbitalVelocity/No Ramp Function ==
  Ain : Inport
  Action Port : ActionPort
  Aout : Outport
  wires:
  Ain/1 -> Aout/1

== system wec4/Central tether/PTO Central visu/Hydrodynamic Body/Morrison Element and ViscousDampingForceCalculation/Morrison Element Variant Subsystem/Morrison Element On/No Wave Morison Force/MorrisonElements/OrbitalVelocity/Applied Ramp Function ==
  Ain : Inport
  Action Port : ActionPort
  Add : Sum
  Constant : Constant  Value=2
  Constant1 : Constant
  Divide : Product  Inputs=**/
  Sine Wave : Sin  Frequency=pi/simu.rampTime  Phase=pi+pi/2  SampleTime=0
  Aout : Outport
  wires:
  Add/1 -> Divide/2
  Sine Wave/1 -> Add/2
  Constant1/1 -> Add/1
  Constant/1 -> Divide/3
  Divide/1 -> Aout/1
  Ain/1 -> Divide/1

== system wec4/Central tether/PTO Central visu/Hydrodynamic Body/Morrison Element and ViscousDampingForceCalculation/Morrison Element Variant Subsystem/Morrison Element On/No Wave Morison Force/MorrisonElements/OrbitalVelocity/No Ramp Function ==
  Ain : Inport
  Action Port : ActionPort
  Aout : Outport
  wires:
  Ain/1 -> Aout/1

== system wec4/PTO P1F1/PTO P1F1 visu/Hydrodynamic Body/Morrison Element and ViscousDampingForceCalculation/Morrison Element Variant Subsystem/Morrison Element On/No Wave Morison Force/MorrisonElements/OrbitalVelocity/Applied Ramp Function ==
  Ain : Inport
  Action Port : ActionPort
  Add : Sum
  Constant : Constant  Value=2
  Constant1 : Constant
  Divide : Product  Inputs=**/
  Sine Wave : Sin  Frequency=pi/simu.rampTime  Phase=pi+pi/2  SampleTime=0
  Aout : Outport
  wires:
  Add/1 -> Divide/2
  Sine Wave/1 -> Add/2
  Constant1/1 -> Add/1
  Constant/1 -> Divide/3
  Divide/1 -> Aout/1
  Ain/1 -> Divide/1

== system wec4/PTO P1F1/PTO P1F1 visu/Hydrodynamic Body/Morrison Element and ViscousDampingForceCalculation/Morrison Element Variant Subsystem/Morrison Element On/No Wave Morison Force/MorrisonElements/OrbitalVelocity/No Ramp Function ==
  Ain : Inport
  Action Port : ActionPort
  Aout : Outport
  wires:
  Ain/1 -> Aout/1

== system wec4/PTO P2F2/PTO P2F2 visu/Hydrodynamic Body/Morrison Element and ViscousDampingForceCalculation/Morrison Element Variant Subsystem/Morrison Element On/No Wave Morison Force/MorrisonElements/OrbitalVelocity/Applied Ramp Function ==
  Ain : Inport
  Action Port : ActionPort
  Add : Sum
  Constant : Constant  Value=2
  Constant1 : Constant
  Divide : Product  Inputs=**/
  Sine Wave : Sin  Frequency=pi/simu.rampTime  Phase=pi+pi/2  SampleTime=0
  Aout : Outport
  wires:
  Add/1 -> Divide/2
  Sine Wave/1 -> Add/2
  Constant1/1 -> Add/1
  Constant/1 -> Divide/3
  Divide/1 -> Aout/1
  Ain/1 -> Divide/1

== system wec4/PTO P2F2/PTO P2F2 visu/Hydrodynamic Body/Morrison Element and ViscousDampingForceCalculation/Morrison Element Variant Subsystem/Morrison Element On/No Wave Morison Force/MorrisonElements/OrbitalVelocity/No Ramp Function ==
  Ain : Inport
  Action Port : ActionPort
  Aout : Outport
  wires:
  Ain/1 -> Aout/1

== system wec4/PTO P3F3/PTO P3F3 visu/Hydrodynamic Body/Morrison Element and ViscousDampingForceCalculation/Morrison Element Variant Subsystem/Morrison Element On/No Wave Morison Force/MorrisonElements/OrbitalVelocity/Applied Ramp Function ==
  Ain : Inport
  Action Port : ActionPort
  Add : Sum
  Constant : Constant  Value=2
  Constant1 : Constant
  Divide : Product  Inputs=**/
  Sine Wave : Sin  Frequency=pi/simu.rampTime  Phase=pi+pi/2  SampleTime=0
  Aout : Outport
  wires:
  Add/1 -> Divide/2
  Sine Wave/1 -> Add/2
  Constant1/1 -> Add/1
  Constant/1 -> Divide/3
  Divide/1 -> Aout/1
  Ain/1 -> Divide/1
